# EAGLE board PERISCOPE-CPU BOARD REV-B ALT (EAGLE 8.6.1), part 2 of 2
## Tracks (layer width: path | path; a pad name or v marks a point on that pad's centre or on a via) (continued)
GND (continued)
  Top 1.016: (E7).7 191.77,132.07 193.09,130.75 193.09,128.33 191.77,127.01 (E6).7 191.77,111.75 193.09,110.43 193.09,108.01 191.77,106.69 (E5).7 191.77,91.43 193.09,90.11 193.09,87.69 191.77,86.37 (E4).7 191.77,69.84 193.09,68.52 193.09,66.1 191.77,64.78 (E3).7 191.77,48.25 193.09,46.93 193.09,44.51 191.77,43.19 (E2).7 191.77,29.21 | 191.77,29.21 (E1).10 | (F8).7 228.6,152.39 229.92,151.07 229.92,148.65 228.6,147.33 (F7).7 228.6,139.33 229.97,137.96 229.97,128.38 228.6,127.01 (F6).7 228.6,111.75 229.92,110.43 229.92,108.01 228.6,106.69 (F5).7 228.6,91.43 229.92,90.11 229.92,87.69 228.6,86.37 (F4).7 228.6,69.84 229.92,68.52 229.92,66.1 228.6,64.78 (F3).7 228.6,48.25 229.92,46.93 229.92,44.51 228.6,43.19 (F2).7 228.6,26.66 229.92,25.34 229.92,22.92 228.6,21.6 (F1).7 228.6,3.17 | (G8).7 266.7,152.39 268.02,151.07 268.02,148.65 266.7,147.33 (G7).7 266.7,132.07 268.02,130.75 268.02,128.33 266.7,127.01 (G6).7 266.7,113.02 268.02,111.7 268.02,109.28 266.7,107.96 (G5).7 266.7,3.17 267.34,3.17 | 191.77,29.21 191.77,26.66 193.09,25.34 193.09,15.3 193.04,15.25 193.04,3.17 | 153.67,29.21 153.67,26.66 154.99,25.34 154.99,3.76 155.57,3.17 | 116.89,30.53 116.89,3.17 116.84,3.17
  Top 2.54: 267.34,3.17 228.6,3.17 193.04,3.17 155.57,3.17 116.84,3.17 77.47,3.17 40.64,3.17 13.34,3.17 13.34,74.6 P1.22 P1.21 5.78,74.44 13.35,74.44 13.55,82.25 13.55,155.24 13.35,155.44 5.78,155.44 P1.2 P1.1
  Bottom 0.152: 185.42,179.07 C5.2 | T1.E 185.42,179.07 | 185.42,179.07 184.2,179.07 179.17,184.1 D5.A | T2.E 185.57,171.6 172.92,171.6 171.55,170.23 R29.1 | R14.1 205.84,143.41 192.89,143.41 191.82,142.34 (E7).7 | R9.1 171.4,167.64 167.59,163.83 156.16,163.83 154.94,162.61 (D8).7
GREEN  (via drill 0.35)
  Top 0.152: v6.2,104.7 6.2,105.61 5.59,106.22 P1.R
  Bottom 0.152: 8.64,104.7 7.11,106.22 5.59,106.22 P1.R | 8.64,104.7 14.28,99.06 115.01,99.06 120.34,104.39 230.68,104.39 233.88,101.19 254.76,101.19 256.44,102.87 (G5).3 | 8.64,104.7 v6.2,104.7
HBLANK  (via drill 0.35)
  Top 0.152: JP12.1 66.09,209.55 66.09,211.99 JP12.2 66.09,212.14 66.09,214.58 JP12.3 66.09,214.73 66.09,217.17 | 66.09,217.17 66.09,219.61 JP12.5 66.09,219.76 66.09,222.2 JP12.6 | 66.09,217.17 JP12.4 | (A3).5 35.61,59.59 37.14,58.06 39.73,58.06 39.73,66.29 40.64,67.21 (A3).8 | v29.06,207.87 29.06,173.28 28.3,172.52 28.3,112.17 30.43,110.03 30.43,67.36 (A3).12
  Bottom 0.152: (A3).12 32.11,65.68 39.12,65.68 40.64,67.21 (A3).8 | v29.06,207.87 64.26,207.87 65.94,209.55 JP12.1
HRESET  (via drill 0.35)
  Top 0.152: v174.14,61.27 174.29,61.11 174.29,21.34 179.02,16.61 (E1).2 | 62.28,217.17 62.28,219.61 JP11.5 62.28,219.76 62.28,222.2 JP11.6 | 62.28,217.17 62.28,214.73 JP11.3 62.28,214.58 62.28,212.14 JP11.2 62.28,211.99 62.28,209.55 JP11.1 62.13,209.55 57.4,204.83 57.4,111.1 57.71,110.8 v57.71,61.27 | 62.28,217.17 JP11.4 | v68.38,25.45 68.38,58.52 67.31,59.59 (B3).3 | v96.27,24.23 v96.27,18.14
  Bottom 0.152: (E1).3 181.61,16.61 179.17,16.61 (E1).2 177.5,14.94 145.03,14.94 143.51,16.46 (D1).3 143.51,16.61 141.07,16.61 (D1).2 140.92,16.61 139.4,18.14 v96.27,18.14 | v174.14,61.27 152.65,61.27 151.13,59.74 (D3).6 | v68.38,25.45 68.68,25.76 92.3,25.76 93.83,24.23 v96.27,24.23 100.23,24.23 (C1).14 | v57.71,61.27 65.79,61.27 67.31,59.74 (B3).3
HSYNC  (via drill 0.35)
  Top 0.152: 69.9,217.17 69.9,219.61 JP13.5 69.9,219.76 69.9,222.2 JP13.6 | v60.15,19.05 60.15,199.95 69.75,209.55 JP13.1 69.9,209.55 69.9,211.99 JP13.2 69.9,212.14 69.9,214.58 JP13.3 69.9,214.73 69.9,217.17 | 69.9,217.17 JP13.4
  Bottom 0.152: v60.15,19.05 35.46,19.05 33.02,16.61 (A1).4
JOYDOWN  (via drill 0.35)
  Top 0.152: 210.87,217.17 210.87,219.61 JP66.5 210.87,219.76 210.87,222.2 JP66.6 | 210.87,217.17 210.87,214.73 JP66.3 210.87,214.58 210.87,212.14 JP66.2 210.87,211.99 210.87,209.55 JP66.1 210.72,209.55 205.84,204.67 v205.84,138.84 | 210.87,217.17 JP66.4 | v5.59,139.6 5.59,138.07 P1.F
  Bottom 0.152: v205.84,138.84 205.54,138.53 184.96,138.53 184.35,137.92 5.59,137.92 P1.F 5.59,138.07 v5.59,139.6
JOYUP  (via drill 0.35)
  Top 0.152: JP65.1 207.06,209.55 207.06,211.99 JP65.2 207.06,212.14 207.06,214.58 JP65.3 207.06,214.73 207.06,217.17 | 207.06,217.17 207.06,219.61 JP65.5 207.06,219.76 207.06,222.2 JP65.6 | 207.06,217.17 JP65.4 | v16.26,142.04 v16.26,210.46 | v5.59,143.56 5.59,142.04 P1.E
  Bottom 0.152: v16.26,210.46 16.41,210.62 205.84,210.62 206.91,209.55 JP65.1 | 5.59,142.04 v16.26,142.04 | 5.59,142.04 v5.59,143.56 | 5.59,142.04 P1.E
N$1
  Bottom 0.152: C1.1 248.97,11.43 250.19,12.65 Q1.2
N$2
  Top 0.152: C1.2 233.73,11.43 233.73,15.24 R2.1
  Bottom 0.152: (F1).4 221.08,16.46 222.61,14.94 233.27,14.94 233.58,15.24 R2.1
N$3
  Top 0.152: R1.1 242.57,21.64 238.76,17.83 C2.1 | (F2).2 214.99,37.19 214.99,17.53 215.9,16.61 (F1).2
  Bottom 0.152: (F2).2 (F2).1 | C2.1 238.76,17.83 238.45,18.14 220.62,18.14 219.41,16.92 219.41,14.94 217.42,14.94 215.9,16.46 (F1).2
N$4
  Bottom 0.152: 233.73,22.55 238.45,22.55 C2.2 | 233.73,22.55 224.43,22.55 218.49,16.61 (F1).3 | 233.73,22.55 233.73,25.3 R2.2
N$5
  Bottom 0.152: Q1.1 250.19,17.68 247.75,15.24 R1.2 241.66,14.33 215.59,14.33 213.46,16.46 (F1).1
N$6
  Bottom 0.152: (E2).12 183.59,43.74 212.7,43.74 218.34,38.1 (F2).3
N$7
  Top 0.152: (E2).1 176.58,38.1 179.02,40.54 179.02,45.72 (E2).13
  Bottom 0.152: R3.2 171.55,49.53 173.69,47.4 177.34,47.4 179.02,45.72 (E2).13 | (E2).4 184.05,38.1 182.37,36.42 178.26,36.42 176.58,38.1 (E2).1
N$8
  Bottom 0.152: 191.67,45.72 189.99,44.04 185.88,44.04 184.2,45.72 (E2).11 | 191.67,45.72 195.48,49.53 R4.2 | 191.67,45.72 (E2).8
N$10  (via drill 0.35)
  Top 0.152: (G8).11 259.03,170.23 259.03,171.75 253.54,171.75 253.09,171.3 253.09,169.16 253.39,168.86 253.39,163.22 254,162.61 (G8).2 v254,160.32 | v193.8,160.32 v193.8,168.71
  Bottom 0.152: v193.8,168.71 170.94,168.71 170.18,167.94 35.31,167.94 31.8,171.45 (A8).12 | v254,160.32 v193.8,160.32
N$11  (via drill 0.35)
  Top 0.152: v152.5,58.06 152.81,57.76 152.81,46.48 153.57,45.72 (D2).8
  Bottom 0.152: (D3).2 142.6,58.06 v152.5,58.06
N$15
  Top 0.152: R7.1 108,54.71 108,59.59 (C3).4
  Bottom 0.152: (C3).4 106.32,58.06 101.91,58.06 100.38,59.59 (C3).1
N$16
  Top 0.152: R8.1 62.28,54.71 62.28,59.59 (B3).1
N$17
  Top 0.152: (B3).2 67.31,57.15 (B2).12
N$19
  Top 0.152: (A4).8 40.95,87.94 40.95,80.92 37.14,77.11 37.14,63.86 33.02,59.74 (A3).4
N$20
  Top 0.152: (A3).3 29.52,60.66 29.52,68.28 30.12,68.89 30.12,87.94 29.21,88.85 (A4).13
N$22
  Bottom 0.152: (A1).5 35.61,16.61 37.44,18.44 65.48,18.44 67.31,16.61 (B1).3
N$28
  Bottom 0.152: (E3).1 181.91,65.08 226.42,65.08 228.55,67.21 (F3).8
N$29
  Top 0.152: (E4).1 178.1,79.7 178.1,60.66 (E3).2
N$33  (via drill 0.35)
  Top 0.152: v31.8,139.14 31.8,143.41 (A7).3
  Bottom 0.152: v31.8,139.14 149.3,139.14 (D7).7
N$35
  Top 0.152: 103.89,125.42 105.41,126.95 (C6).12 | 103.89,125.42 100.38,121.92 (C6).1 | 103.89,125.42 103.89,141.28 102.97,142.19 (C7).2
N$38
  Top 0.152: (F4).4 222.61,82.91 222.61,108.2 223.52,109.12 (F5).10
N$39
  Top 0.152: (F5).12 217.42,108.2 217.42,80.31 218.03,79.7 223.52,79.7 (F4).5
N$95
  Top 0.152: R31.2 Q2.C
N$96
  Top 0.152: (F7).12 223.52,144.78 (F7).5
N$97
  Top 0.152: (F6).5 223.52,124.51 218.49,129.54 (F6).12
N$98
  Top 0.152: (F4).3 218.49,81.38 220.01,82.91 220.01,100.58 220.93,101.5 (F5).4 221.08,101.65 222.15,102.72 222.15,120.85 221.08,121.92 (F6).4
  Bottom 0.152: (F5).4 219.41,103.17 214.99,103.17 213.46,101.65 (F5).1
N$99  (via drill 0.35)
  Top 0.152: v214.53,131.22 214.22,131.52 214.22,141.43 | 214.22,141.43 213.46,142.19 (F7).1 | 214.22,141.43 214.22,148.13 215.9,149.81 (F7).13
  Bottom 0.152: v214.53,131.22 224.28,131.22 225.96,129.54 (F6).9 | D3.C 199.44,156.21 204.16,151.49 214.38,151.49 215.9,149.96 (F7).13
N$100
  Top 0.152: (F7).4 221.08,142.19 221.54,141.73 SW1.P$1
  Bottom 0.152: SW1.P$1 R5.1
N$101  (via drill 0.35)
  Top 0.152: v230.99,149.81 v230.99,103.17 | D4.C 171.25,158.95 v171.25,158.65
  Bottom 0.152: v230.99,103.17 225.04,103.17 223.52,101.65 (F5).5 | v230.99,149.81 228.7,149.81 (F7).8 228.55,149.96 227.03,151.49 222.3,151.49 215.14,158.65 v171.25,158.65
N$102
  Top 0.152: (F5).6 226.11,101.5 226.11,96.62 R28.1
N$103
  Top 0.152: R30.2 171.4,172.82 171.4,175.26 R31.1
  Bottom 0.152: D4.A 167.74,172.82 171.4,172.82 R30.2
N$104
  Top 0.152: (E5).3 181.61,101.65 183.13,103.17 183.13,121.01 184.05,121.92 (E6).4
  Bottom 0.152: (D5).4 155.25,103.17 180.09,103.17 181.61,101.65 (E5).3
N$105  (via drill 0.35)
  Top 0.152: v200.66,110.8 200.66,165.05 199.44,166.27 D3.A
  Bottom 0.152: T2.C 195.48,169.01 195.48,167.64 R33.1 195.63,167.64 196.39,166.88 198.83,166.88 199.29,166.42 D3.A | v200.66,110.8 224.43,110.8 225.96,109.27 (F5).9
N$106
  Top 0.152: C4.2 R32.1 R33.2 185.42,168.71 181.46,168.71 180.54,169.62 180.54,177.7 179.17,179.07 Q2.B
N$107
  Top 0.152: R29.2 R30.1 181.61,172.82 184.05,175.26 C5.1 | T2.B 189.23,176.63 191.67,179.07 T1.C
  Bottom 0.152: C5.1 186.79,175.26 189.23,172.82 T2.B
N$108  (via drill 0.35)
  Top 0.152: v188.01,127.86 188.32,127.56 188.32,102.56 189.23,101.65 (E5).6
  Bottom 0.152: (E6).12 183.29,127.86 v188.01,127.86
N$109  (via drill 0.35)
  Top 0.152: v153.72,161.24 153.72,109.27 (D5).5
  Bottom 0.152: v153.72,161.24 154.03,160.93 179.93,160.93 180.24,161.24 C6.1
N$112
  Bottom 0.152: (E6).3 179.93,123.6 143.97,123.6 142.29,121.92 (D6).2
N$114
  Top 0.152: (D6).1 140,121.62 140,116.74 147.47,109.27 147.47,105.31 151.13,101.65 (D5).3
N$115
  Bottom 0.152: (G6).3 256.59,121.92 264.21,129.54 (G6).9
N$116  (via drill 0.35)
  Top 0.152: v239.98,111.4 239.98,186.69 C7.1
  Bottom 0.152: 151.13,109.27 148.69,109.27 (D5).7 | R35.2 C7.1 | 151.13,109.27 153.26,111.4 v239.98,111.4 | 151.13,109.27 (D5).6
N$117
  Top 0.152: (G6).10 264.06,127.1 264.06,121.92 (G6).6
N$118
  Top 0.152: VR1.2 R35.1
  Bottom 0.152: VR1.3 256.44,179.07 VR1.2
N$119
  Bottom 0.152: (F4).6 226.11,81.38 229.77,85.04 234.95,85.04 D1.A
N$120
  Top 0.152: (F6).1 213.46,121.92 215.9,124.36 (F6).13 215.9,133.35 R37.1
N$121
  Top 0.152: (G5).2 259.03,107.9 259.03,110.49 (G5).11
N$122
  Bottom 0.152: (G5).1 251.56,102.87 257.5,108.81 264.97,108.81 266.65,110.49 (G5).8
N$123
  Bottom 0.152: (F7).2 215.9,142.19 213,139.29 208.13,139.29 207.06,138.23 189.08,138.23 186.79,135.94 R38.1
N$125
  Top 0.152: 65.79,125.42 67.31,126.95 (B6).12 | 65.79,125.42 62.28,121.92 (B6).1 | 65.79,125.42 65.79,141.28 64.87,142.19 (B7).2
N$126
  Bottom 0.152: (A5).8 43.23,107.9 61.52,107.9 61.82,107.59 63.19,107.59 64.72,109.12 (B5).13
N$127  (via drill 0.35)
  Top 0.152: v188.32,160.02 188.32,143.26 189.23,142.34 (E7).6
  Bottom 0.152: v188.32,160.02 188.01,160.32 169.11,160.32 168.81,160.63 144.73,160.63 143.2,162.15 143.2,164.13 141.22,164.13 139.7,162.61 (D8).1
N$128  (via drill 0.35)
  Top 0.152: v72.49,131.52 72.49,142.19 (B7).5
  Bottom 0.152: v72.49,131.52 74.47,129.54 (B6).9
N$129
  Top 0.152: (B7).10 71.42,148.9 71.42,128.47 72.03,127.86 77.37,127.86 77.37,129.54 (B6).8
N$130
  Top 0.152: (B7).13 64.87,149.81 68.83,145.85 68.83,130.45 69.75,129.54 (B6).11
N$131
  Top 0.152: 111.81,127.86 111.81,128.32 (C6).9 | 111.81,127.86 111.81,121.31 103.89,113.39 103.89,102.56 102.97,101.65 (C5).2 | (C7).5 109.52,141.28 109.52,128.47 110.13,127.86 111.81,127.86
N$133  (via drill 0.35)
  Top 0.152: v111.05,131.67 111.51,132.13 111.51,148.9 110.59,149.81 (C7).10
  Bottom 0.152: v111.05,131.67 111.51,131.22 113.79,131.22 115.47,129.54 (C6).8
N$134  (via drill 0.35)
  Top 0.152: v97.03,127.86 v97.03,101.65 | (C7).13 102.97,149.81 106.93,145.85 106.93,130.45 107.85,129.54 (C6).11
  Bottom 0.152: v97.03,101.65 100.23,101.65 (C5).1 | v97.03,127.86 106.17,127.86 107.85,129.54 (C6).11
N$135
  Bottom 0.152: (A7).1 29.52,140.66 65.79,140.66 67.31,142.19 (B7).3
N$136  (via drill 0.35)
  Top 0.152: v74.93,145.69 (B7).6
  Bottom 0.152: v74.93,145.69 74.62,145.39 36.22,145.39 34.39,143.56 (A7).4
N$137
  Bottom 0.152: (B7).8 75.23,152.09 42.93,152.09 42.32,152.71 40.95,152.71 (A7).9
N$138
  Bottom 0.152: (C7).3 105.41,142.34 103.58,144.17 44.6,144.17 42.32,141.88 30.73,141.88 29.21,143.41 (A7).2
N$139
  Bottom 0.152: (C7).6 113.03,142.34 110.29,145.09 38.35,145.09 36.83,143.56 (A7).5
N$140  (via drill 0.35)
  Top 0.152: (C7).8 114.4,151.03 v114.4,153.31
  Bottom 0.152: v114.4,153.31 38.96,153.31 36.83,151.18 (A7).10
N$141
  Bottom 0.152: (B7).11 69.75,149.81 68.22,148.28 34.54,148.28 31.8,151.03 (A7).12
N$142  (via drill 0.35)
  Top 0.152: v107.85,153.92 107.85,149.96 (C7).11
  Bottom 0.152: v107.85,153.92 107.54,153.62 31.65,153.62 29.21,151.18 (A7).13
N$143
  Bottom 0.152: (A6).3 31.8,121.92 33.48,123.6 101.14,123.6 102.82,121.92 (C6).2 (C6).3
N$144  (via drill 0.35)
  Top 0.152: v39.42,139.75 39.42,143.41 (A7).6 | v138.63,139.75 137.26,141.12 137.26,142.19 (D7).1
  Bottom 0.152: v138.63,139.75 v39.42,139.75
N$145
  Bottom 0.152: (A7).8 42.01,151.18 42.62,151.79 74.93,151.79 76.45,150.27 76.45,145.39 136.65,145.39 139.7,142.34 (D7).2
N$146  (via drill 0.35)
  Top 0.152: (A7).11 35.31,150.11 v35.31,140.06
  Bottom 0.152: v35.31,140.06 35.61,140.36 147.93,140.36 149.76,142.19 (D7).6
N$147
  Bottom 0.152: (G8).12 254.31,167.94 221.23,167.94 215.9,162.61 (F8).2
N$148
  Bottom 0.152: (F8).3 222.61,166.73 263.3,166.73 266.65,170.08 (G8).8
N$149
  Bottom 0.152: (F8).4 221.08,162.61 222.61,164.13 262.53,164.13 264.06,162.61 (G8).6
N$150  (via drill 0.35)
  Top 0.152: v256.44,160.63 256.44,149.96 (G7).12
  Bottom 0.152: v256.44,160.63 256.13,160.93 225.04,160.93 223.52,162.46 (F8).5
N$151  (via drill 0.35)
  Top 0.152: v227.03,145.24 227.03,161.54 226.11,162.46 (F8).6
  Bottom 0.152: (G7).6 261.16,145.24 v227.03,145.24
N$152  (via drill 0.35)
  Top 0.152: v222,152.71 222,169.16 (F8).11
  Bottom 0.152: v222,152.71 263.91,152.71 266.65,149.96 (G7).8
N$153  (via drill 0.35)
  Top 0.152: v181.61,166.27 (E7).12
  Bottom 0.152: v181.61,166.27 197.31,166.27 198.83,164.74 213,164.74 (F8).12
N$154
  Top 0.152: (D7).3 142.29,142.19 142.29,135.94 R40.1
  Bottom 0.152: (D7).5 147.32,142.34 145.8,143.87 143.81,143.87 142.29,142.34 (D7).3
N$156
  Top 0.152: (F8).1 213.46,162.46 213.46,157.58 R41.1
N$163
  Bottom 0.152: (B8).3 68.99,165.51 102.51,165.51 105.41,162.61 (C8).3
N$170  (via drill 0.35)
  Top 0.152: v258.12,144.63 258.12,161.54 259.03,162.46 (G8).4 | v63.35,152.71 63.35,162.76 62.28,163.83 (B8).1
  Bottom 0.152: 255.83,144.17 256.29,144.63 v258.12,144.63 | 255.83,144.17 254,142.34 (G7).2 | v63.35,152.71 63.65,152.4 172.01,152.4 180.54,143.87 196.24,143.87 196.39,143.71 212.4,143.71 212.85,144.17 255.83,144.17
N$174  (via drill 0.35)
  Top 0.152: v40.34,134.42 40.34,162.92 39.42,163.83 (A8).6
  Bottom 0.152: v40.34,134.42 187.25,134.42 188.62,135.79 207.67,135.79 210.57,138.68 258.12,138.68 261.62,142.19 (G7).5
N$177
  Bottom 0.152: (D8).2 142.29,162.46 144.42,160.32 168.66,160.32 179.02,149.96 (E7).13 179.02,149.81 178.71,149.81 178.71,146.15 179.02,145.85 255.07,145.85 (G7).11
N$211
  Bottom 0.152: (B5).5 67.31,106.68 36.83,106.68 (A5).11
N$213
  Top 0.152: 186.64,129.54 186.64,129.39 179.17,121.92 (E6).2 | 186.64,129.54 186.64,133.35 R47.1 | 186.64,129.54 (E6).10
OCEAN  (via drill 0.35)
  Top 0.152: 148.69,209.55 148.69,211.99 JP52.2 148.69,212.14 148.69,214.58 JP52.3 148.69,214.73 148.69,217.17 | 148.69,217.17 148.69,219.61 JP52.5 148.69,219.76 148.69,222.2 JP52.6 | 148.69,217.17 JP52.4 | v180.7,106.98 180.7,82.3 181.61,81.38 (E4).3 | (G6).12 256.44,129.54 255.52,128.63 255.52,111.4 256.44,110.49 (G5).12 | 148.69,209.55 148.84,209.4 148.84,110.49 149.76,109.58 v149.76,106.98 | 148.69,209.55 JP52.1
  Bottom 0.152: (G5).12 256.44,110.49 253.24,107.29 181,107.29 v180.7,106.98 v149.76,106.98
ONES  (via drill 0.35)
  Top 0.152: v35.31,111.1 35.31,102.56 34.39,101.65 (A5).4
  Bottom 0.152: v35.31,111.1 75.54,111.1 77.37,109.27 (B5).8
P1LED  (via drill 0.35)
  Top 0.152: v5.59,115.82 5.59,114.3 P1.N | 191.82,217.17 191.82,219.61 JP61.5 191.82,219.76 191.82,222.2 JP61.6 | 191.82,209.55 191.82,211.99 JP61.2 191.82,212.14 191.82,214.58 JP61.3 191.82,214.73 191.82,217.17 | v194.41,96.62 v194.41,114.3 194.41,206.96 191.82,209.55 | 191.82,209.55 JP61.1 | 191.82,217.17 JP61.4
  Bottom 0.152: 5.59,114.3 v5.59,115.82 | v194.41,96.62 215.9,96.62 R28.2 | v194.41,114.3 5.59,114.3 | 5.59,114.3 P1.N
Q  (via drill 0.35)
  Top 0.152: (F5).8 227.63,110.19 227.63,123.44 222.61,128.47 222.61,130.61 224.43,132.44 224.43,148.9 223.52,149.81 (F7).10 | 179.17,217.17 179.17,219.61 JP60.5 179.17,219.76 179.17,222.2 JP60.6 | 179.17,217.17 179.17,214.73 JP60.3 179.17,214.58 179.17,212.14 JP60.2 179.17,211.99 179.17,209.55 JP60.1 179.02,209.55 177.8,208.33 177.8,131.98 178.26,131.52 178.26,128.78 | 179.17,217.17 JP60.4 | (E5).1 178.26,103.33 v178.26,107.59 178.26,108.05 177.8,108.51 177.8,128.32 178.26,128.78 | 178.26,128.78 179.02,129.54 (E6).13
  Bottom 0.152: v178.26,107.59 227.03,107.59 228.55,109.12 (F5).8
RED  (via drill 0.35)
  Top 0.152: v265.58,112.78 265.58,128.47 266.65,129.54 (G6).8 | v5.59,111.86 5.59,110.34 P1.P
  Bottom 0.152: v265.58,112.78 8.03,112.78 7.11,111.86 | 7.11,111.86 5.59,110.34 P1.P | 7.11,111.86 v5.59,111.86
SCORE  (via drill 0.35)
  Top 0.152: 199.44,217.17 199.44,219.61 JP63.5 199.44,219.76 199.44,222.2 JP63.6 | v228.55,208.48 228.55,170.23 (F8).8 | (G6).5 257.81,125.73 257.81,144.02 252.78,149.05 v252.78,168.55 | JP63.1 199.44,209.55 199.44,211.99 JP63.2 199.44,212.14 199.44,214.58 JP63.3 199.44,214.73 199.44,217.17 | 199.44,217.17 JP63.4
  Bottom 0.152: v228.55,208.48 200.51,208.48 199.44,209.55 JP63.1 | v252.78,168.55 230.23,168.55 (F8).8
SCOREEN  (via drill 0.35)
  Top 0.152: v144.73,132.28 144.73,142.19 (D7).4
  Bottom 0.152: v144.73,132.28 38.35,132.28 38.35,128.63 39.12,127.86 40.18,127.86 41.86,129.54 (A6).8
SCOREVEN  (via drill 0.35)
  Top 0.152: (C5).8 114.4,108.05 v114.4,99.67
  Bottom 0.152: 35.31,99.97 30.73,99.97 29.21,101.5 (A5).2 | 35.31,99.97 36.83,101.5 (A5).5 | v114.4,99.67 35.61,99.67 35.31,99.97
SOUND  (via drill 0.35)
  Top 0.152: 203.25,217.17 203.25,219.61 JP64.5 203.25,219.76 203.25,222.2 JP64.6 | 203.25,217.17 203.25,214.73 JP64.3 203.25,214.58 203.25,212.14 JP64.2 203.25,211.99 203.25,209.55 JP64.1 203.1,209.55 202.03,208.48 v202.03,85.19 | 203.25,217.17 JP64.4 | v5.59,84.89 5.59,86.41 P1.19
  Bottom 0.152: v202.03,85.19 5.89,85.19 v5.59,84.89
START  (via drill 0.35)
  Top 0.152: 163.93,217.17 163.93,219.61 JP56.5 163.93,219.76 163.93,222.2 JP56.6 | 163.93,209.55 v163.93,127.25 | 163.93,209.55 163.93,211.99 JP56.2 163.93,212.14 163.93,214.58 JP56.3 163.93,214.73 163.93,217.17 | 163.93,209.55 JP56.1 | 163.93,217.17 JP56.4
  Bottom 0.152: 63.04,120.24 28.45,120.24 26.77,121.92 (A6).1 | 63.04,120.24 64.72,121.92 (B6).2 (B6).3 | (E6).9 188.62,128.93 188.62,127.25 v163.93,127.25 163.32,126.64 109.52,126.64 109.52,121.46 108.31,120.24 63.04,120.24
SUBMARINE  (via drill 0.35)
  Top 0.152: (G5).10 259.94,112.17 257.5,112.17 257.5,109.42 256.9,108.81 254.91,108.81 254.91,121.01 (G6).2 | JP54.1 156.31,209.55 156.31,211.99 JP54.2 156.31,212.14 156.31,214.58 JP54.3 156.31,214.73 156.31,217.17 | 156.31,217.17 156.31,219.61 JP54.5 156.31,219.76 156.31,222.2 JP54.6 | 156.31,217.17 JP54.4 | 197.92,146.15 197.92,135.79 196.85,134.72 R16.2 | 197.92,146.15 196.85,147.22 R12.2 | 197.92,146.15 v197.92,208.48
  Bottom 0.152: v197.92,208.48 157.38,208.48 156.31,209.55 JP54.1 | (G6).2 248.36,127.56 203.25,127.56 196.85,133.96 R16.2
SYNC  (via drill 0.35)
  Top 0.152: JP51.1 144.88,209.55 144.88,211.99 JP51.2 144.88,212.14 144.88,214.58 JP51.3 144.88,214.73 144.88,217.17 | 144.88,217.17 144.88,219.61 JP51.5 144.88,219.76 144.88,222.2 JP51.6 | 144.88,217.17 JP51.4 | v37.14,98.3 37.14,90.68 37.74,90.07 37.74,80.16 36.83,79.25 36.83,66.6 32.11,61.87 32.11,22.55 38.05,16.61 (A1).6 | v129.64,98.3 v129.64,209.55 | v5.59,99.97 5.59,98.45 P1.T
  Bottom 0.152: v129.64,209.55 JP51.1 | v129.64,98.3 v37.14,98.3 5.59,98.3 P1.T 5.59,98.45 v5.59,99.97
TENS
  Bottom 0.152: (A5).1 26.77,101.65 28.3,103.17 57.1,103.17 60.3,99.97 73.41,99.97 74.93,101.5 (B5).6
TORPEDO  (via drill 0.35)
  Top 0.152: 160.12,209.55 160.12,211.99 JP55.2 160.12,212.14 160.12,214.58 JP55.3 160.12,214.73 160.12,217.17 | 160.12,217.17 160.12,219.61 JP55.5 160.12,219.76 160.12,222.2 JP55.6 | 160.12,217.17 JP55.4 | R13.2 R14.2 R15.2 196.85,139.6 195.78,138.53 195.78,134.11 196.7,133.2 v198.53,133.2 | (G5).13 253.09,111.4 253.09,128.63 (G6).13 254,131.22 256.9,131.22 257.5,130.61 257.5,123.44 259.03,121.92 (G6).4 | v160.12,139.6 160.12,209.55 | 160.12,209.55 JP55.1
  Bottom 0.152: v198.53,133.2 250.34,133.2 (G6).13 | v160.12,139.6 196.85,139.6 R15.2
VBLANK  (via drill 0.35)
  Top 0.152: JP37.6 JP37.5 JP37.4 JP37.3 JP37.2 JP37.1 123.39,208.48 v123.39,77.57 | (A4).1 26.77,81.23 26.92,81.08 26.92,41.61 30.43,38.1 (A2).3
  Bottom 0.152: (A2).4 (A2).3 | v123.39,77.57 123.09,77.88 30.12,77.88 26.77,81.23 (A4).1
VCC  (via drill 0.35)
  Top 0.152: 176.58,95.25 R34.2 | 176.53,135.79 176.58,135.79 R38.2 | 176.58,133.35 R47.2 | (F6).10 227.33,133.35 R37.2 227.33,136.55 227.94,137.16 SW1.P$2 | v211.63,157.58 211.86,157.58 | v195.63,157.58 195.63,165.05 R32.2 | (E7).14 176.58,150.27 176.58,179.07 Q2.E
  Top 1.016: (A8).14 26.67,166.36 25.35,165.04 25.35,162.62 26.67,161.3 (A7).14 26.67,146.04 25.35,144.72 25.35,142.3 26.67,140.98 (A6).14 26.67,124.45 25.35,123.13 25.35,120.71 26.67,119.39 (A5).14 26.67,104.13 25.35,102.81 25.35,100.39 26.67,99.07 (A4).14 26.67,83.81 25.35,82.49 25.35,80.07 25.4,80.02 (A3).14 25.4,62.22 24.08,60.9 24.08,58.48 25.4,57.16 (A2).14 25.4,40.63 24.08,39.31 24.08,36.89 25.4,35.57 (A1).14 | (B1).14 62.23,35.57 60.91,36.89 60.91,39.31 62.23,40.63 (B2).14 | 62.23,46.36 (B2).14 | (B2).14 62.23,52.74 60.91,54.06 60.91,60.9 62.23,62.22 (B3).14 62.23,78.75 60.91,80.07 60.91,82.49 62.23,83.81 (B4).14 62.23,99.07 60.91,100.39 60.91,102.81 62.23,104.13 (B5).14 | (B5).14 62.23,111.76 (B6).5 | (B5).14 62.23,119.39 60.91,120.71 60.91,143.45 62.23,144.77 (B7).14 62.23,161.3 60.91,162.62 60.91,165.04 62.23,166.36 (B8).14 | (C8).14 100.33,165.09 99.01,163.77 99.01,161.35 100.33,160.03 (C7).14 100.33,144.77 99.01,143.45 99.01,120.71 100.33,119.39 (C5).14 | (C5).14 100.33,111.76 (C6).5 | (C5).14 100.33,104.13 99.01,102.81 99.01,100.39 100.33,99.07 (C4).14 100.33,83.81 99.01,82.49 99.01,80.07 100.33,78.75 (C3).14 100.33,62.22 99.01,60.9 99.01,58.48 100.33,57.16 100.33,48.25 99.01,46.93 99.01,35.56 | (C1).5 104.85,22.15 99.78,22.15 99.01,22.92 99.01,35.56 | (C2).5 110.48,38.1 108.5,36.12 99.57,36.12 99.01,35.56 | (D1).5 142.95,22.15 137.88,22.15 137.11,22.92 137.11,39.31 138.43,40.63 (D2).14 138.43,57.16 137.11,58.48 137.11,60.9 138.43,62.22 (D3).14 138.43,78.75 137.11,80.07 137.11,82.49 138.43,83.81 (D4).14 138.43,101.6
  Top 1.016: 138.43,101.6 (D5).8 | 138.43,101.6 138.43,120.66 138.38,120.71 138.38,123.13 139.7,124.45 (D6).14 139.7,137.17 135.84,141.03 135.84,143.45 137.16,144.77 (D7).16 137.16,167.64 (D8).14 | (E7).14 176.53,144.77 175.21,143.45 175.21,141.03 176.53,139.71 R38.2 176.53,135.79 R47.2 (E6).14 176.53,124.45 175.21,123.13 175.21,120.71 176.53,119.39 (E5).14 176.53,104.13 175.21,102.81 175.21,100.39 176.53,99.07 R34.2 (E4).14 176.53,83.81 175.21,82.49 175.21,80.07 176.53,78.75 (E3).14 176.53,62.22 175.21,60.9 175.21,55.26 176.58,53.89 176.58,52.79 176.53,52.74 (E2).14 176.53,40.63 175.21,39.31 175.21,22.92 175.98,22.15 181.05,22.15 (E1).5 | (F1).14 213.36,35.57 212.04,36.89 212.04,39.31 213.36,40.63 (F2).14 213.36,57.16 212.04,58.48 212.04,60.9 213.36,62.22 (F3).14 213.36,78.75 212.04,80.07 212.04,82.49 213.36,83.81 (F4).14 213.36,99.07 212.04,100.39 212.04,102.81 213.36,104.13 (F5).14 213.36,119.39 212.04,120.71 212.04,123.13 213.36,124.45 (F6).14 213.36,139.71 212.04,141.03 212.04,143.45 213.36,144.77 (F7).14 213.36,155.36 211.86,156.86 211.86,157.58 211.86,163.59 213.36,165.09 (F8).14 | (G8).14 251.46,165.09 250.14,163.77 250.14,161.35 251.46,160.03 (G7).14 251.46,144.77 250.14,143.45 250.14,141.03 251.46,139.71 (G6).14 251.46,124.45 250.14,123.13 250.14,120.71 251.46,119.39 (G5).14
  Bottom 0.152: R40.2 152.5,135.94 176.43,135.94 R38.2 | C4.1 188.01,161.39 191.67,165.05 195.48,165.05 R32.2 | Q2.E 163.63,179.07 162.78,179.92 | v211.63,157.58 203.25,157.58 R41.2 203.1,157.58 v195.63,157.58 | (F6).10 221.84,127.86 215.14,127.86 213.46,129.54 (F6).14
  Bottom 1.016: VR1.1 251.46,175.9 | 251.46,175.9 (G8).14 | 243.84,175.9 251.46,175.9 | (F8).14 213.36,175.9 | (D8).14 139.7,177.16 | (C8).14 100.33,177.16 | (B8).14 62.23,177.16 | (A8).14 26.67,177.16
  Bottom 2.54: P1.C P1.D 14.61,145.92 14.61,177.16 26.67,177.16 62.23,177.16 100.33,177.16 139.7,177.16 160.02,177.16 162.78,179.92 175.26,192.41 194.94,192.41 211.45,175.9 213.36,175.9 243.84,175.9
VRESET  (via drill 0.35)
  Top 0.152: JP36.6 JP36.5 JP36.4 JP36.3 JP36.2 JP36.1 121.72,208.48 v121.72,39.78 | v74.02,40.39 74.02,58.67 74.93,59.59 (B3).6 | v97.94,40.08 97.94,22.86 99.01,21.79 99.01,20.42 102.82,16.61 (C1).2
  Bottom 0.152: (C1).2 102.97,16.61 105.41,16.61 (C1).3 | 74.02,40.08 v97.94,40.08 100.84,40.08 101.14,39.78 | 74.02,40.08 29.97,40.08 27.99,38.1 (A2).2 | 101.14,39.78 102.82,38.1 (C2).2 (C2).3 | 74.02,40.08 v74.02,40.39 | 101.14,39.78 v121.72,39.78
VSYNC  (via drill 0.35)
  Top 0.152: JP38.6 JP38.5 JP38.4 JP38.3 JP38.2 JP38.1 127.2,208.48 v127.2,19.96
  Bottom 0.152: v127.2,19.96 31.34,19.96 27.99,16.61 (A1).2

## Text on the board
Top: PERISCOPE - CPU | 13 | 27 | 38 | 51 | 60 | 61 | 70 | 1 | REV - B | (c) KINCAIDARCADE 2018 | KincaidArcade.com | 26 | 39 | 14 | 50 | 8 | 7 | 6 | 5 | 4 | 3 | Engineered By: / ALEXANDER H. | (A 15 Year Old!) | 2 | 1 | D | E | F | G | B | C | A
